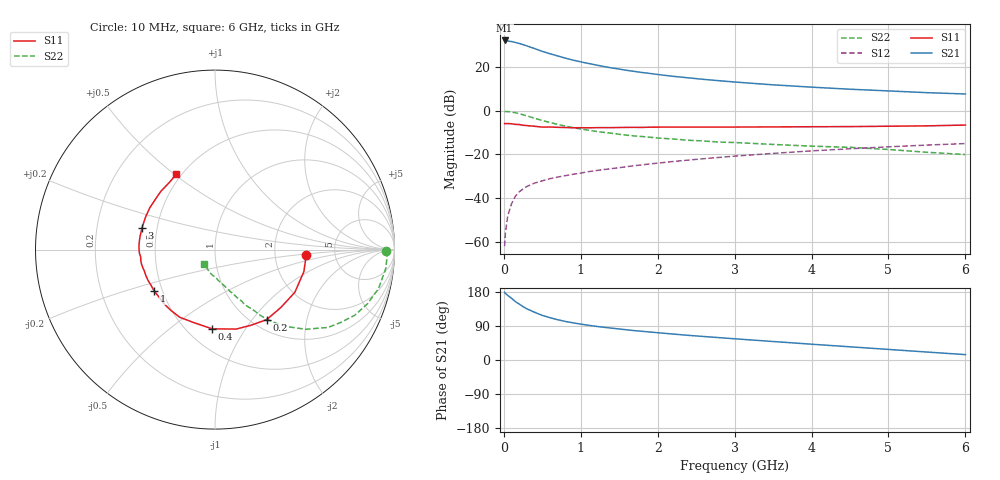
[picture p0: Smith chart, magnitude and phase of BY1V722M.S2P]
! SIEMENS Small Signal Semiconductors
! BFY420
! Si NPN RF SIEGET Grounded Emitter Transistor in MICRO-X
! VCE = 1.75 V  IC = 22 mA
! Common Emitter S-Parameters:  October  1996
# GHz  S  MA  R  50
!  f  S11  S21  S12  S22
! GHz  MAG  ANG  MAG  ANG  MAG  ANG  MAG  ANG
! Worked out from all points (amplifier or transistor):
!   36 points, 10 MHz to 6 GHz, reference 50 ohm
!   highest |S21| = 32.2 dB at 10 MHz (marker M1)
!   |S21| within 3 dB of that: start of sweep to 340.9 MHz
!   unconditionally stable (mu >= 1): 1.785 GHz to end of sweep
!   at 250 MHz: K = 0.32, MSG = 33.0 dB, |S12| = -35.8 dB
!   at 1.4 GHz: K = 0.93, MSG = 23.0 dB, |S12| = -26.5 dB
!   at 6 GHz: K = 1.08, MAG = 9.6 dB, |S12| = -15.0 dB
!   S11 on the Smith chart (normalised r, x): 10 MHz: 3.05, -0.23; 200 MHz: 1.16, -1.18; 400 MHz: 0.66, -0.72; 1 GHz: 0.45, -0.25; 3 GHz: 0.41, +0.12; 6 GHz: 0.47, +0.51
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0.01  0.5089 -3.1  40.59 178.6  0.0008 102.7  0.9517 -0.6
0.02  0.5079 -6.3  40.3 175.6  0.0016 85.4  0.9596 -2.1
0.05  0.5102 -13.9  39.26 170.7  0.0039 83.1  0.9574 -6.3
0.1  0.5045 -28.2  38.36 162.9  0.0075 80.2  0.9367 -13.4
0.15  0.4885 -41.3  36.49 154.1  0.0111 72.9  0.9009 -19.7
0.2  0.4848 -53.6  34.74 147.6  0.014 70.1  0.8599 -25.2
0.25  0.4667 -64.7  32.52 140.7  0.0163 66.4  0.8085 -30.2
0.3  0.4581 -75.1  30.43 135.0  0.0186 64.8  0.7651 -34.5
0.4  0.4419 -92.0  26.44 125.9  0.0222 60.9  0.674 -41.2
0.5  0.4237 -105.9  22.84 117.7  0.025 59.1  0.5983 -46.1
0.6  0.4251 -117.5  20.16 111.6  0.028 58.0  0.538 -50.0
0.7  0.4183 -126.4  17.95 106.3  0.0305 57.3  0.4876 -53.1
0.8  0.4144 -133.7  15.98 101.8  0.0328 56.9  0.4455 -55.4
1  0.4097 -145.9  13.15 94.7  0.0376 57.6  0.384 -58.7
1.1  0.4082 -151.4  12.11 91.6  0.0405 57.7  0.3599 -60.6
1.6  0.4171 -168.6  8.401 79.5  0.0527 57.1  0.2764 -66.8
2.2  0.4243 177.4  6.142 68.5  0.0691 55.5  0.2265 -73.0
3  0.4244 163.4  4.55 56.0  0.0917 51.1  0.1879 -79.8
3.5  0.4273 155.0  3.919 48.8  0.106 47.8  0.1699 -84.6
4.5  0.4345 139.9  3.112 34.8  0.1352 39.4  0.146 -94.0
5.5  0.4522 124.4  2.596 21.0  0.1642 30.1  0.1124 -112.7
6  0.4711 117.3  2.422 14.2  0.1777 25.0  0.0997 -127.2
